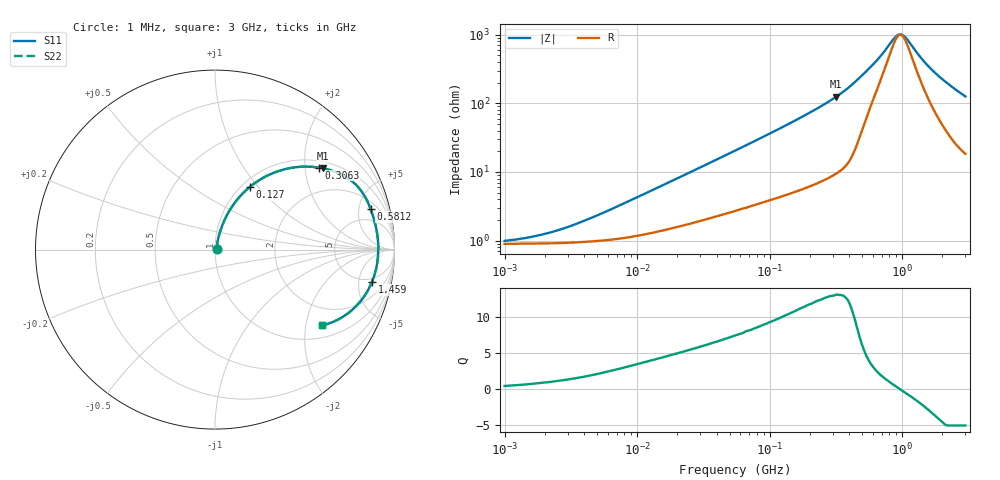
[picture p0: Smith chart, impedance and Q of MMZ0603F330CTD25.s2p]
! S-parameter Generated by TDK Corporation
! Copyright(C) 2018 TDK Corporation.
! All Rights Reserved.
! TDK P/N: MMZ0603F330CTD25 (Chip Bead)
! Property: |Z|=33¶ at 100MHz
! Size(LxWxT): 0.6x0.3x0.3mm, 0.024x0.012x0.012inches
! Model Type: s2p (Touchstone File Format Version 1.0)
! Frequency: DC=Yes Start=1MHz Stop=3000MHz 202points Log-sweep
! Model Generated on Aug. 6, 2018
! Port Assignments:
!  1 ---@@@--- 2
! Applicable Conditions:
!  Temperature = 25 degC
!  DC Bias Current = 0 A
!  Small Signal Operation
! Terms and conditions regarding TDK Simulation Models
! (1)This simulation model is being provided solely for informational purposes. Please refer to the specifications of the products in terms of detailed characteristics of such products.
! (2)In no event shall TDK Corporation of any of its subsidiaries be liable for any loss or damage arising, directly or indirectly,
!  From any information contained in this simulation model, including, but not limited to loss or damages arising from any inaccuracies, omissions or errors in connection with such information.
! (3)Any and all copyrights on this simulation model are owned by TDK Corporation.
!  Duplication or redistribution of this simulation model without prior written permission from TDK Corporation is prohibited.
! (4)This simulation model is subject to any modification or change without any prior notice.
! (5)Neither TDK Corporation nor any of its subsidiaries shall make any warranty, express or implied,
!  Including but not limited to the correctness, implied warranties of merchantability and fitness for a particular purpose with respect to this simulation models.
! (6)The use of this simulation model shall be deemed to have consented to the terms and conditions hereof.
# Hz S MA R 50
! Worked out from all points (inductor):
!   201 points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, 1 MHz to 3 GHz, reference 50 ohm
!   read as one part in series: L = 65.7 nH near 8.018 MHz
!   highest Q = 13.1 at 318.8 MHz (marker M1), where L = 62.2 nH
!   self-resonance near 969.4 MHz
!   S11 on the Smith chart (normalised r, x): 1 MHz: 1.02, +0.01; 127 MHz: 1.09, +0.91; 306.3 MHz: 1.18, +2.37; 581.2 MHz: 2.86, +6.56; 1.459 GHz: 4.22, -7.50; 3 GHz: 1.37, -2.49
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1000000  0.009854 25.3  0.9911 -0.2  0.9911 -0.2  0.009854 25.3
1974946  0.01233 42.4  0.9909 -0.5  0.9909 -0.5  0.01233 42.4
3900413  0.01895 59.1  0.9904 -0.9  0.9904 -0.9  0.01895 59.1
1.461624e7  0.05958 73.6  0.9848 -3.3  0.9848 -3.3  0.05958 73.6
3.00453e7  0.114 74.0  0.9747 -6.5  0.9747 -6.5  0.114 74.0
5.477226e7  0.1951 71.2  0.9553 -11.1  0.9553 -11.1  0.1951 71.2
8.854986e7  0.297 66.4  0.9224 -17.2  0.9224 -17.2  0.297 66.4
1.269575e8  0.4011 60.8  0.8774 -23.5  0.8774 -23.5  0.4011 60.8
2.136344e8  0.5922 49.1  0.7582 -36.2  0.7582 -36.2  0.5922 49.1
3.062963e8  0.7374 38.3  0.6214 -47.3  0.6214 -47.3  0.7374 38.3
3.188066e8  0.7532 37.0  0.6031 -48.7  0.6031 -48.7  0.7532 37.0
4.219165e8  0.8525 26.6  0.45 -58.1  0.45 -58.1  0.8525 26.6
4.951867e8  0.8833 20.3  0.3506 -60.7  0.3506 -60.7  0.8833 20.3
5.81181e8  0.8957 14.6  0.2628 -59.5  0.2628 -59.5  0.8957 14.6
6.821091e8  0.9029 9.8  0.1886 -54.3  0.1886 -54.3  0.9029 9.8
8.005644e8  0.9079 5.3  0.127 -41.0  0.127 -41.0  0.9079 5.3
8.672962e8  0.9095 3.1  0.1038 -27.8  0.1038 -27.8  0.9095 3.1
9.395906e8  0.91 0.9  0.09112 -8.6  0.09112 -8.6  0.91 0.9
1.017911e9  0.9095 -1.4  0.0933 13.4  0.0933 13.4  0.9095 -1.4
1.45942e9  0.8932 -11.6  0.2189 55.2  0.2189 55.2  0.8932 -11.6
2.01032e9  0.8476 -21.7  0.3785 55.9  0.3785 55.9  0.8476 -21.7
3e9  0.7321 -35.2  0.5823 46.4  0.5823 46.4  0.7321 -35.2
